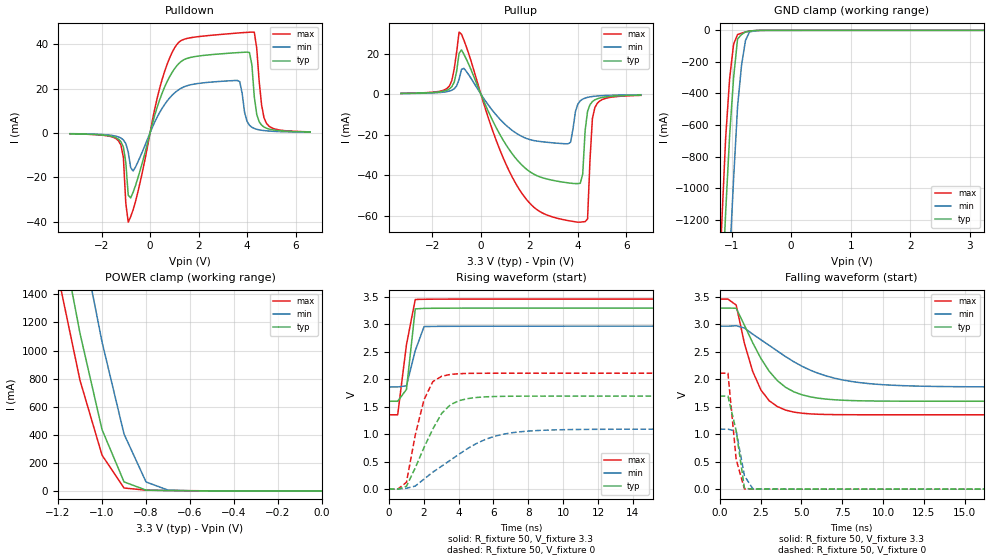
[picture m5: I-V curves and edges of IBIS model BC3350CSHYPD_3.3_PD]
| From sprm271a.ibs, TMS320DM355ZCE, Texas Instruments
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|   GS50 Cell BC3350CSHYPD
|   Model Cell BC3350CSHYPD_3.3_PD
[Model]   BC3350CSHYPD_3.3_PD
Model_type   I/O
Polarity   Non-Inverting
Enable   Active-Low
Vinl =  1.5
Vinh =  1.8
Cref =  15.0000pF
Rref =  100.0000M
Vref =  0V
Vmeas =  1.65
C_comp   0.972592p   0.9599789p   0.9808023p
[Model Spec]
Vinl   1.5   1.335   1.5825
Vinh   1.8   1.635   1.8825
[Temperature Range]   25   125   -40
[Voltage Range]   3.3   2.97   3.465
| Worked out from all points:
|   slope of the pulldown table from 0 to 0.495 V, typ, clamps not added: 27.7 ohm
|   slope of the pullup table from 0 to 0.495 V, typ, clamps not added: 37.2 ohm
|   GND clamp passes 1 mA (typ) near -0.58 V on its own axis
|   POWER clamp passes 1 mA (typ) near -0.54 V on its own axis
|   rising waveform, R_fixture 50, V_fixture 3.3: 20-80 % time 351ps typ, 605ps min, 589ps max; typ from 1.6 V to 3.3 V
|   rising waveform, R_fixture 50, V_fixture 0: 20-80 % time 1.55ns typ, 3.16ns min, 923ps max; typ from 0 V to 1.7 V
|   falling waveform, R_fixture 50, V_fixture 3.3: 20-80 % time 2.12ns typ, 3.92ns min, 1.37ns max; typ from 3.3 V to 1.6 V
|   falling waveform, R_fixture 50, V_fixture 0: 20-80 % time 583ps typ, 447ps min, 479ps max; typ from 1.7 V to 0 V
[POWER_clamp]
|   voltage   I(typ)   I(min)   I(max)
-3.3V     22.26A     22.97A     21.87A
-1.2V     1.947A     2.724A     1.536A
-1.167V   1.672A     2.436A     1.287A
-1.133V   1.397A     2.148A     1.037A
-1.1V     1.122A     1.86A      787.1mA
-1.067V   893.3mA    1.594A     609.6mA
-1.033V   665.2mA    1.327A     432.1mA
-1V       437mA      1.061A     254.5mA
-900mV    64.23mA    405.2mA    20.86mA
-800mV    5.876mA    63.96mA    5.368mA
-700mV    2.696mA    5.798mA    3.296mA
-11.55fV  98.21uA    49.4uA     162.3uA
[Pulldown]
|   voltage   I(typ)   I(min)   I(max)
-3.3V     -403.6uA   -328.8uA   -418.9uA
-1.3V     -2.841mA   -1.807mA   -3.581mA
-1.1V     -6.386mA   -3.145mA   -10.99mA
-900mV    -28.11mA   -8.625mA   -40.3mA
-700mV    -26.82mA   -17.2mA    -34.77mA
400mV     15.05mA    9.288mA    20.3mA
1.1V      30.25mA    18.85mA    39.86mA
3.7V      36.3mA     23.15mA    45.16mA
4.2V      30.69mA    2.555mA    45.51mA
4.4V      8.338mA    1.643mA    38.15mA
4.8V      2.127mA    941.5uA    4.342mA
6.6V      435.4uA    314uA      481.3uA
[Pullup]
|   voltage   I(typ)   I(min)   I(max)
-3.3V     327.4uA    259.3uA    367uA
-1.3V     2.541mA    1.473mA    3.994mA
-900mV    20.05mA    7.198mA    30.58mA
-700mV    19.65mA    12.69mA    26.57mA
1.6V      -33.88mA   -20.32mA   -47.31mA
3.6V      -43.79mA   -24.49mA   -62.4mA
4.1V      -44.01mA   -3.32mA    -63.19mA
4.2V      -39.34mA   -2.47mA    -63.02mA
4.4V      -8.445mA   -1.612mA   -61.59mA
4.6V      -3.699mA   -1.188mA   -11.99mA
4.7V      -2.851mA   -1.049mA   -6.684mA
6.6V      -510.5uA   -319.6uA   -632.9uA
[GND_clamp]
|   voltage   I(typ)   I(min)   I(max)
-3.3V     -22.38A    -23.15A    -21.96A
-1.167V   -1.724A    -2.574A    -1.236A
-1.1V     -1.155A    -1.991A    -683mA
-1.033V   -667.4mA   -1.447A    -306.4mA
-966.7mV  -300.8mA   -944.1mA   -87.56mA
-900mV    -54.72mA   -483.8mA   -26.56mA
-833.3mV  -26.41mA   -221.5mA   -17.75mA
-766.7mV  -9.715mA   -63.74mA   -10.4mA
-700mV    -4.628mA   -10.65mA   -4.496mA
-566.7mV  -735.2uA   -1.508mA   -502.4uA
-433.3mV  -74.69uA   -170.3uA   -70.93uA
3.233V    98.2uA     61.67uA    162.2uA
[Ramp]
| variable   typ   min   max
dV/dt_f   1.029523/2.114981n   0.6729414/3.944544n   1.277356/1.372726n
dV/dt_r   1.01722/1.522676n   0.6557512/3.142093n   1.267173/0.9091869n
R_load = 50
[Rising Waveform]
R_fixture = 50
V_fixture = 3.3
V_fixture_min = 2.97
V_fixture_max = 3.465
| time   V(typ)   V(min)   V(max)
|   time   V(typ)   V(min)   V(max)
0s        1.601V     1.861V     1.354V
505.1ps   1.601V     1.861V     1.354V
1.01ns    1.817V     1.882V     2.632V
1.515ns   3.283V     2.523V     3.455V
2.02ns    3.293V     2.961V     3.458V
50ns      3.298V     2.969V     3.462V
[Rising Waveform]
R_fixture = 50
V_fixture = 0
V_fixture_min = 0
V_fixture_max = 0
| time   V(typ)   V(min)   V(max)
|   time   V(typ)   V(min)   V(max)
0s        57.79nV    466.6nV    5.374nV
505.1ps   -6.176uV   122.1nV    -260.7uV
1.01ns    52.58mV    17.06mV    124.2mV
1.515ns   388.1mV    56.33mV    986.7mV
2.02ns    760.9mV    184mV      1.632V
2.525ns   1.098V     310mV      1.959V
3.535ns   1.539V     528.3mV    2.09V
6.061ns   1.688V     962.5mV    2.111V
9.091ns   1.695V     1.076V     2.112V
50ns      1.695V     1.092V     2.112V
[Falling Waveform]
R_fixture = 50
V_fixture = 3.3
V_fixture_min = 2.97
V_fixture_max = 3.465
| time   V(typ)   V(min)   V(max)
|   time   V(typ)   V(min)   V(max)
0s        3.298V     2.969V     3.462V
1.01ns    3.295V     2.976V     3.352V
1.515ns   2.985V     2.935V     2.653V
2.02ns    2.667V     2.823V     2.144V
2.525ns   2.38V      2.72V      1.806V
3.535ns   1.975V     2.515V     1.504V
4.545ns   1.772V     2.319V     1.403V
7.576ns   1.619V     1.986V     1.356V
11.62ns   1.602V     1.881V     1.354V
50ns      1.601V     1.861V     1.354V
[Falling Waveform]
R_fixture = 50
V_fixture = 0
V_fixture_min = 0
V_fixture_max = 0
| time   V(typ)   V(min)   V(max)
|   time   V(typ)   V(min)   V(max)
0s        1.695V     1.092V     2.112V
505.1ps   1.695V     1.092V     2.112V
1.01ns    1.062V     1.055V     538.2mV
1.515ns   14.91mV    244.2mV    3.398mV
2.02ns    2.31mV     9.645mV    1.345mV
2.525ns   1.308mV    2.361mV    701.8uV
50ns      106.2nV    504nV      39.07nV
